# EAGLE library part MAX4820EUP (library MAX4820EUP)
Gate Drivers +3.3V/+5V, 8-Channel, Cascadable Relay Drivers with Serial/Parallel Interface Source: Datasheet
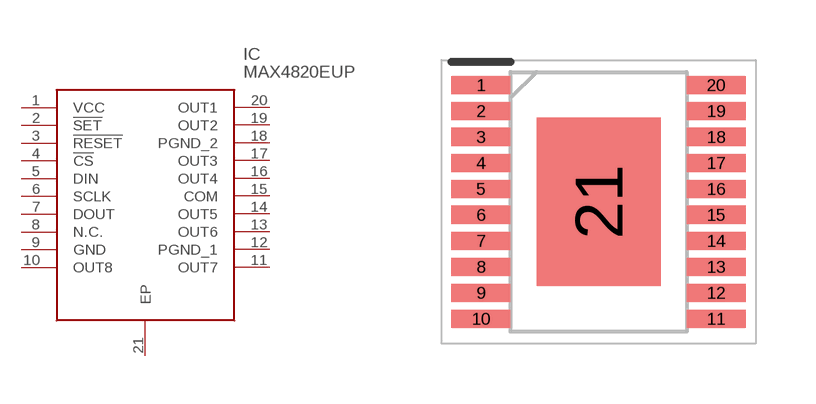
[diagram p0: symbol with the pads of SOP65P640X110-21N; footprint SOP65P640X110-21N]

Designator prefix IC

## MAX4820EUP (Description: Gate Drivers +3.3V/+5V, 8-Channel, Cascadable Relay Drivers with Serial/Parallel Interface; Height: 1.1mm; Manufacturer_Name: Maxim Integrated; Manufacturer_Part_Number: MAX4820EUP; Mouser_Part_Number: N/A; Mouser_Price-Stock: https://www.mouser.com/Search/Refine.aspx?Keyword=N%2FA)  [SOP65P640X110-21N]
1  VCC
2  !SET
3  !RESET
4  !CS
5  DIN
6  SCLK
7  DOUT
8  N.C.  nc
9  GND
10  OUT8
11  OUT7
12  PGND_1
13  OUT6
14  OUT5
15  COM
16  OUT4
17  OUT3
18  PGND_2
19  OUT2
20  OUT1
21  EP

## Footprint SOP65P640X110-21N (pad centres in mm)
TSSOP 20 pin
smd 1.475 x 0.45: 1 -2.938,2.925; 2 -2.938,2.275; 3 -2.938,1.625; 4 -2.938,0.975; 5 -2.938,0.325; 6 -2.938,-0.325; 7 -2.938,-0.975; 8 -2.938,-1.625; 9 -2.938,-2.275; 10 -2.938,-2.925; 11 2.938,-2.925; 12 2.938,-2.275; 13 2.938,-1.625; 14 2.938,-0.975; 15 2.938,-0.325; 16 2.938,0.325; 17 2.938,0.975; 18 2.938,1.625; 19 2.938,2.275; 20 2.938,2.925
smd 3.1 x 4.2: 21 0,0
